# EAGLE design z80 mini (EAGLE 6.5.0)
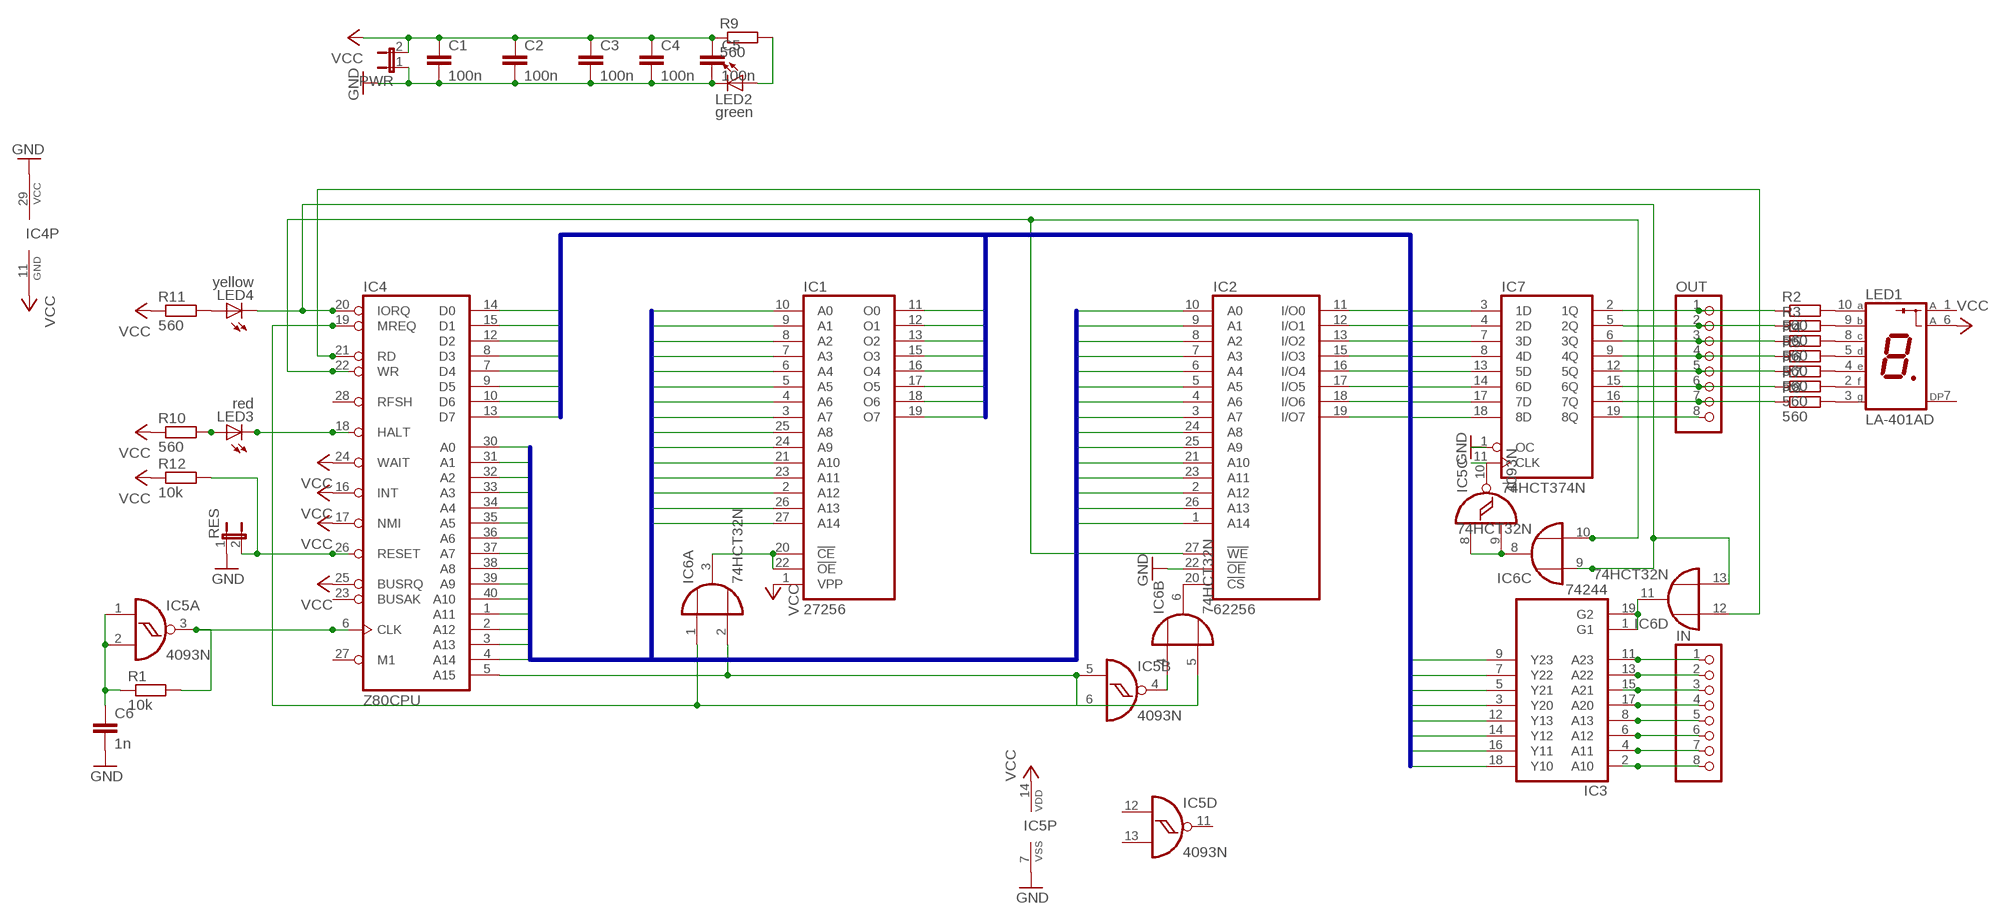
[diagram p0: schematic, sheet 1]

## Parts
C1  100n  C-EU025-025X050  [C025-025X050]
C2  100n  C-EU025-025X050  [C025-025X050]
C3  100n  C-EU025-025X050  [C025-025X050]
C4  100n  C-EU025-025X050  [C025-025X050]
C5  100n  C-EU025-025X050  [C025-025X050]
C6  1n  C-EU025-025X050  [C025-025X050]
IC1  27256  [DIL28]
IC2  62256  [DIL28]
IC3  74244  [DIL20]
IC4  Z80CPU  [DIL40]
IC5  4093N  [DIL14]
IC6  74HCT32N  [DIL14]
IC7  74HCT374N  [DIL20]
IN  PINHD-1X8  [1X08]
LED1  LA-401AD  [LA-401]
LED2  green  LED3MM  [LED3MM]
LED3  red  LED3MM  [LED3MM]
LED4  yellow  LED3MM  [LED3MM]
OUT  PINHD-1X8  [1X08]
PWR  JP1E  [JP1]
R1  10k  R-EU_0204/7  [0204/7]
R2  560  R-EU_0204/7  [0204/7]
R3  560  R-EU_0204/7  [0204/7]
R4  560  R-EU_0204/7  [0204/7]
R5  560  R-EU_0204/7  [0204/7]
R6  560  R-EU_0204/7  [0204/7]
R7  560  R-EU_0204/7  [0204/7]
R8  560  R-EU_0204/7  [0204/7]
R9  560  R-EU_0204/7  [0204/7]
R10  560  R-EU_0204/7  [0204/7]
R11  560  R-EU_0204/7  [0204/7]
R12  10k  R-EU_0204/7  [0204/7]
RES  JP1E  [JP1]

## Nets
A0: IC1.10(A0) IC2.10(A0) IC4.30(A0)
A1: IC1.9(A1) IC2.9(A1) IC4.31(A1)
A2: IC1.8(A2) IC2.8(A2) IC4.32(A2)
A3: IC1.7(A3) IC2.7(A3) IC4.33(A3)
A4: IC1.6(A4) IC2.6(A4) IC4.34(A4)
A5: IC1.5(A5) IC2.5(A5) IC4.35(A5)
A6: IC1.4(A6) IC2.4(A6) IC4.36(A6)
A7: IC1.3(A7) IC2.3(A7) IC4.37(A7)
A8: IC1.25(A8) IC2.24(A8) IC4.38(A8)
A9: IC1.24(A9) IC2.25(A9) IC4.39(A9)
A10: IC1.21(A10) IC2.21(A10) IC4.40(A10)
A11: IC1.23(A11) IC2.23(A11) IC4.1(A11)
A12: IC1.2(A12) IC2.2(A12) IC4.2(A12)
A13: IC1.26(A13) IC2.26(A13) IC4.3(A13)
A14: IC1.27(A14) IC2.1(A14) IC4.4(A14)
D0: IC1.11(O0) IC2.11(I/O0) IC3.18(Y10) IC4.14(D0) IC7.3(1D)
D1: IC1.12(O1) IC2.12(I/O1) IC3.16(Y11) IC4.15(D1) IC7.4(2D)
D2: IC1.13(O2) IC2.13(I/O2) IC3.14(Y12) IC4.12(D2) IC7.7(3D)
D3: IC1.15(O3) IC2.15(I/O3) IC3.12(Y13) IC4.8(D3) IC7.8(4D)
D4: IC1.16(O4) IC2.16(I/O4) IC3.3(Y20) IC4.7(D4) IC7.13(5D)
D5: IC1.17(O5) IC2.17(I/O5) IC3.5(Y21) IC4.9(D5) IC7.14(6D)
D6: IC1.18(O6) IC2.18(I/O6) IC3.7(Y22) IC4.10(D6) IC7.17(7D)
D7: IC1.19(O7) IC2.19(I/O7) IC3.9(Y23) IC4.13(D7) IC7.18(8D)
GND: C1.2 C2.2 C3.2 C4.2 C5.2 C6.2 IC2.22(!OE) IC4.29(VCC) IC5.7(P:VSS) IC7.1(OC) LED2.K(C) PWR.1 RES.1
N$1: C6.1 IC5.1(A:I0) IC5.2(A:I1) R1.1
N$2: IC4.6(CLK) IC5.3(A:O) R1.2
N$3: IC3.11(A23) IN.1
N$4: IC3.13(A22) IN.2
N$5: IC3.15(A21) IN.3
N$6: IC3.17(A20) IN.4
N$7: IC3.8(A13) IN.5
N$8: IC3.6(A12) IN.6
N$9: IC3.4(A11) IN.7
N$10: IC3.2(A10) IN.8
N$11: IC7.2(1Q) OUT.1 R2.1
N$12: IC7.5(2Q) OUT.2 R3.1
N$13: IC7.6(3Q) OUT.3 R4.1
N$14: IC7.9(4Q) OUT.4 R5.1
N$15: IC7.12(5Q) OUT.5 R6.1
N$16: IC7.15(6Q) OUT.6 R7.1
N$17: IC7.16(7Q) OUT.7 R8.1
N$18: IC7.19(8Q) OUT.8
N$19: LED1.10(A) R2.2
N$20: LED1.9(B) R3.2
N$21: LED1.8(C) R4.2
N$22: LED1.5(D) R5.2
N$23: LED1.4(E) R6.2
N$24: LED1.2(F) R7.2
N$25: LED1.3(G) R8.2
N$26: IC5.4(B:O) IC6.4(B:I0)
N$27: IC2.20(!CS) IC6.6(B:O)
N$28: IC1.20(!CE) IC1.22(!OE) IC6.3(A:O)
N$29: IC4.5(A15) IC5.5(B:I0) IC5.6(B:I1) IC6.2(A:I1)
N$30: IC4.19(MREQ) IC6.1(A:I0) IC6.5(B:I1)
N$31: IC2.27(!WE) IC4.22(WR) IC6.10(C:I1)
N$32: IC5.10(C:O) IC7.11(CLK)
N$33: IC5.8(C:I0) IC5.9(C:I1) IC6.8(C:O)
N$34: IC4.20(IORQ) IC6.9(C:I0) IC6.13(D:I1) LED4.K(C)
N$35: IC3.1(G1) IC3.19(G2) IC6.11(D:O)
N$36: IC4.18(HALT) LED3.K(C)
N$37: IC4.21(RD) IC6.12(D:I0)
N$38: LED2.A R9.2
N$39: LED3.A R10.2
N$40: LED4.A R11.2
N$41: IC4.26(RESET) R12.2 RES.2
VCC: C1.1 C2.1 C3.1 C4.1 C5.1 IC1.1(VPP) IC4.11(GND) IC4.16(INT) IC4.17(NMI) IC4.24(WAIT) IC4.25(BUSRQ) IC5.14(P:VDD) LED1.6(A) PWR.2 R9.1 R10.1 R11.1 R12.1
Unconnected: IC4.23(BUSAK) IC4.27(M1) IC4.28(RFSH) IC5.11(D:O) IC5.12(D:I0) IC5.13(D:I1) LED1.1(A) LED1.7(DP)

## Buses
D[0..7]
A[0..14]

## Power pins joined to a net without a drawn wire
GND: IC1.14(GND) IC2.14(GND) IC3.10(GND) IC6.7(P:GND) IC7.10(GND)
VCC: IC1.28(VCC) IC2.28(VCC) IC3.20(VCC) IC6.14(P:VCC) IC7.20(VCC)

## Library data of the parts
C1-C6 = resistor:C-EU: CAPACITOR, European symbol
IC1 = 0RB_Memory:27256: MEMORY
IC2 = 0RB_Memory:62256: 32K*8 SRAM
IC3 = 0RB_TTL:74244: 74244 as one IC
IC4 = 0RB_Zilog:Z80CPU: Z80 CPU
IC5 = 40xx:4093: Quad 2-input NAND schmitt trigger
IC6 = 74xx-eu:74*32: Quad 2-input OR gate
IC7 = 74xx-eu:74*374: Octal D type transparent LATCH, edge triggered
IN OUT = pinhead:PINHD-1X8: PIN HEADER
LED1 = led-7-segment:LA-401*D: Single Digit LED Numeric Display (anode common) Source: ROHM .. la-1401dn.pdf
LED2-LED4 = led:LED: LED
PWR RES = jumper:JP1E: JUMPER
R1-R12 = resistor:R-EU_: RESISTOR, European symbol

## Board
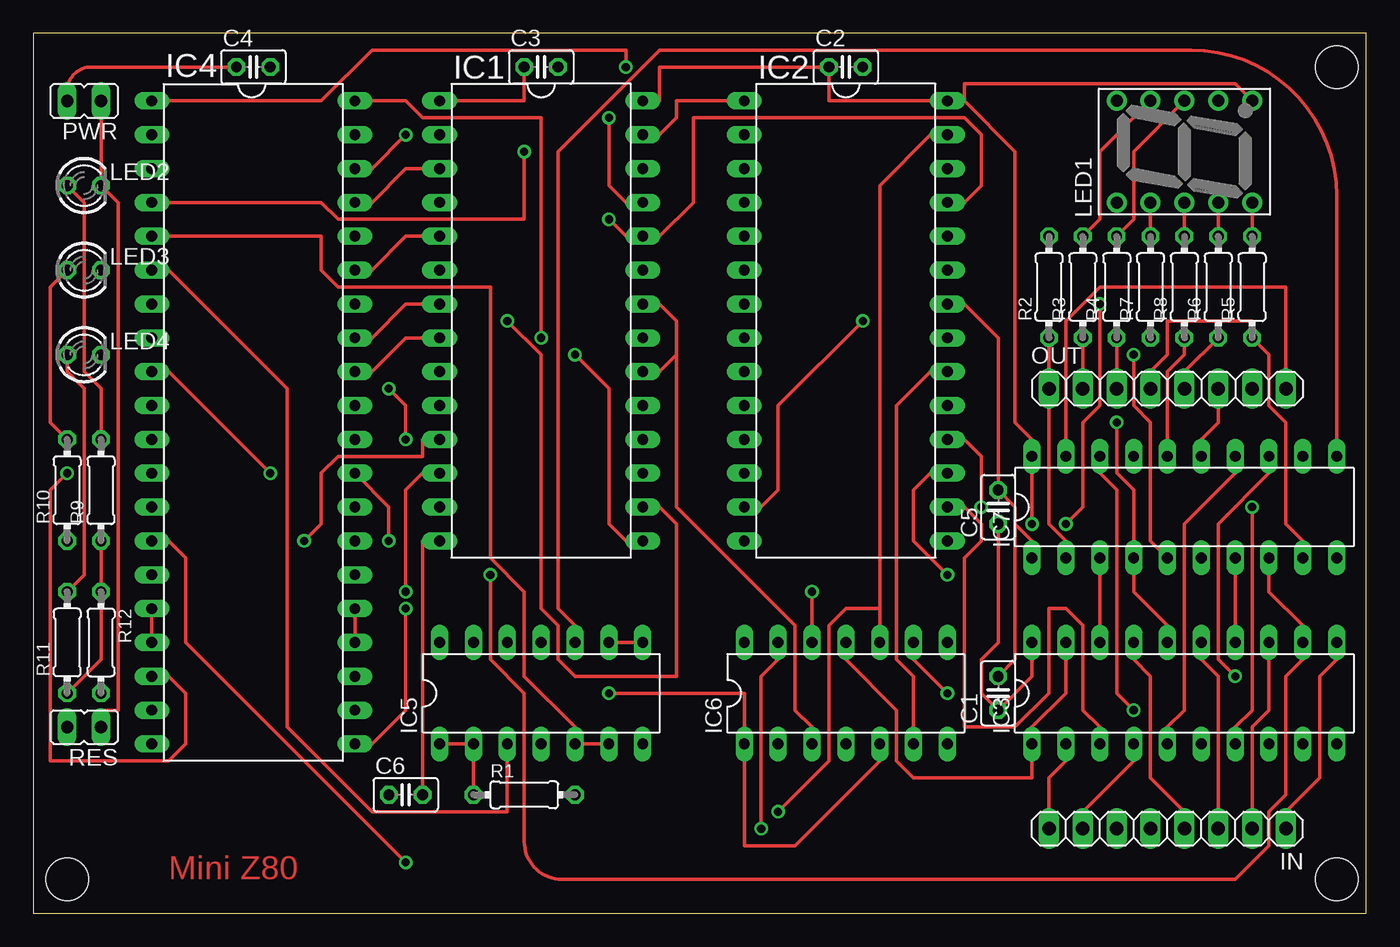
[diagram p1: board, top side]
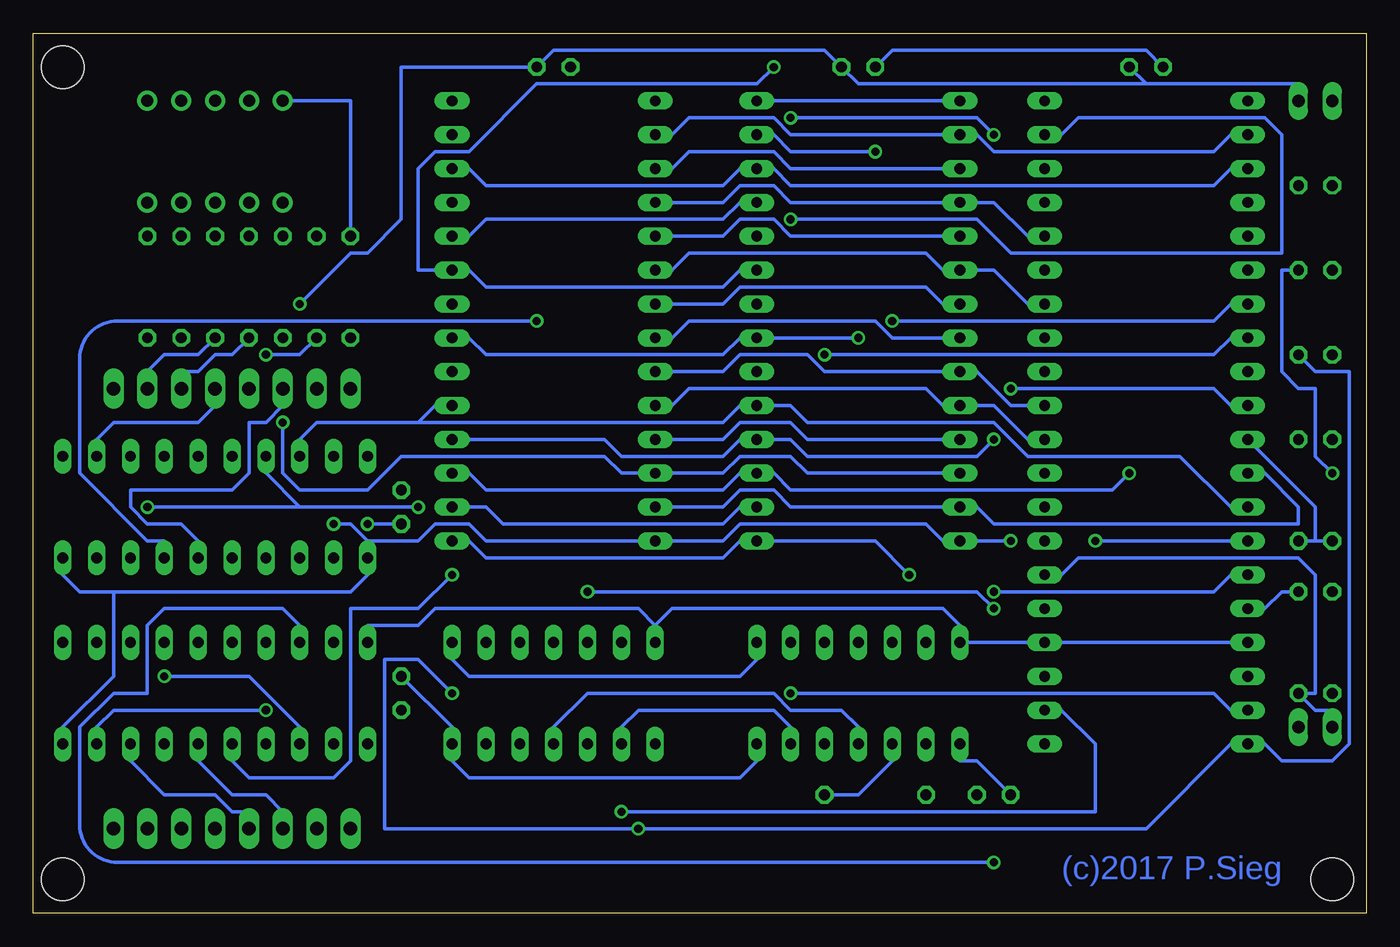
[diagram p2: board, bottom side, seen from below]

Size 100 x 66.03 mm. Coordinates in mm from the lower left corner, seen from the top.
Outline: 0,0 100,0 100,66.03 0,66.03 0,0
Copper layers (1*16): Top 0.035mm / dielectric 1.5mm / Bottom 0.035mm
Design rules "default": minimum track width 10mil, minimum drill 24mil, track to track 8mil, track to pad 8mil, pad to pad 8mil, via to via 8mil, smd to smd 8mil, copper to edge 40mil, drill to drill 8mil, minimum pad ring 10mil, minimum via ring 8mil, stop-mask expansion 4mil, vias tented up to drill 0mil, thermal gap 10mil
Holes 3.2 mm at 2.54,2.54 97.79,63.5 97.79,2.54

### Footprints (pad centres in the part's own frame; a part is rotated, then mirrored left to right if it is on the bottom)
C025-025X050 = drill 0.813 octagon: 1 -1.27,0; 2 1.27,0
DIL28 = drill 0.813 long: 1 -16.51,-7.62; 2 -13.97,-7.62; 3 -11.43,-7.62; 4 -8.89,-7.62; 5 -6.35,-7.62; 6 -3.81,-7.62; 7 -1.27,-7.62; 8 1.27,-7.62; 9 3.81,-7.62; 10 6.35,-7.62; 11 8.89,-7.62; 12 11.43,-7.62; 13 13.97,-7.62; 14 16.51,-7.62; 15 16.51,7.62; 16 13.97,7.62; 17 11.43,7.62; 18 8.89,7.62; 19 6.35,7.62; 20 3.81,7.62; 21 1.27,7.62; 22 -1.27,7.62; 23 -3.81,7.62; 24 -6.35,7.62; 25 -8.89,7.62; 26 -11.43,7.62; 27 -13.97,7.62; 28 -16.51,7.62
DIL20 = drill 0.813 long: 1 -11.43,-3.81; 2 -8.89,-3.81; 3 -6.35,-3.81; 4 -3.81,-3.81; 5 -1.27,-3.81; 6 1.27,-3.81; 7 3.81,-3.81; 8 6.35,-3.81; 9 8.89,-3.81; 10 11.43,-3.81; 11 11.43,3.81; 12 8.89,3.81; 13 6.35,3.81; 14 3.81,3.81; 15 1.27,3.81; 16 -1.27,3.81; 17 -3.81,3.81; 18 -6.35,3.81; 19 -8.89,3.81; 20 -11.43,3.81
DIL40 = drill 0.813 long: 1 -24.13,-7.62; 2 -21.59,-7.62; 3 -19.05,-7.62; 4 -16.51,-7.62; 5 -13.97,-7.62; 6 -11.43,-7.62; 7 -8.89,-7.62; 8 -6.35,-7.62; 9 -3.81,-7.62; 10 -1.27,-7.62; 11 1.27,-7.62; 12 3.81,-7.62; 13 6.35,-7.62; 14 8.89,-7.62; 15 11.43,-7.62; 16 13.97,-7.62; 17 16.51,-7.62; 18 19.05,-7.62; 19 21.59,-7.62; 20 24.13,-7.62; 21 24.13,7.62; 22 21.59,7.62; 23 19.05,7.62; 24 16.51,7.62; 25 13.97,7.62; 26 11.43,7.62; 27 8.89,7.62; 28 6.35,7.62; 29 3.81,7.62; 30 1.27,7.62; 31 -1.27,7.62; 32 -3.81,7.62; 33 -6.35,7.62; 34 -8.89,7.62; 35 -11.43,7.62; 36 -13.97,7.62; 37 -16.51,7.62; 38 -19.05,7.62; 39 -21.59,7.62; 40 -24.13,7.62
DIL14 = drill 0.813 long: 1 -7.62,-3.81; 2 -5.08,-3.81; 3 -2.54,-3.81; 4 0,-3.81; 5 2.54,-3.81; 6 5.08,-3.81; 7 7.62,-3.81; 8 7.62,3.81; 9 5.08,3.81; 10 2.54,3.81; 11 0,3.81; 12 -2.54,3.81; 13 -5.08,3.81; 14 -7.62,3.81
1X08 = drill 1.016 long: 1 -8.89,0; 2 -6.35,0; 3 -3.81,0; 4 -1.27,0; 5 1.27,0; 6 3.81,0; 7 6.35,0; 8 8.89,0
LA-401 = drill 0.9 pad 1.5: 1 -3.81,5.08; 2 -3.81,2.54; 3 -3.81,0; 4 -3.81,-2.54; 5 -3.81,-5.08; 6 3.81,-5.08; 7 3.81,-2.54; 8 3.81,0; 9 3.81,2.54; 10 3.81,5.08
LED3MM = drill 0.813 octagon: A -1.27,0; K 1.27,0
JP1 = drill 0.914 long: 1 0,-1.27; 2 0,1.27
0204/7 = drill 0.813 octagon: 1 -3.81,0; 2 3.81,0

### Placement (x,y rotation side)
C1  72.39,16.51 90 top
C2  60.96,63.5 0 top
C3  38.1,63.5 0 top
C4  16.51,63.5 0 top
C5  72.39,30.48 90 top
C6  27.94,8.89 0 top
IC1  38.1,44.45 270 top
IC2  60.96,44.45 270 top
IC3  86.36,16.51 0 top
IC4  16.51,36.83 270 top
IC5  38.1,16.51 0 top
IC6  60.96,16.51 0 top
IC7  86.36,30.48 0 top
IN  85.09,6.35 180 top
LED1  86.36,57.15 90 top
LED2  3.81,54.61 0 top
LED3  3.81,48.26 0 top
LED4  3.81,41.91 0 top
OUT  85.09,39.37 0 top
PWR  3.81,60.96 90 top
R1  36.83,8.89 0 top
R2  76.2,46.99 90 top
R3  78.74,46.99 90 top
R4  81.28,46.99 90 top
R5  91.44,46.99 90 top
R6  88.9,46.99 90 top
R7  83.82,46.99 90 top
R8  86.36,46.99 90 top
R9  5.08,31.75 90 top
R10  2.54,31.75 90 top
R11  2.54,20.32 90 top
R12  5.08,20.32 270 top
RES  3.81,13.97 90 top

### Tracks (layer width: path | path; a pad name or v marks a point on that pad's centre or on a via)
A0
  Bottom 0.254: IC4.30 25.4,35.56 27.94,38.1 IC1.10 31.75,38.1 33.02,39.37 50.8,39.37 52.07,38.1 IC2.10
A1
  Bottom 0.254: IC4.31 26.67,38.1 29.21,40.64 IC1.9 40.64,40.64 41.91,41.91 46.99,41.91 48.26,40.64 IC2.9
A2
  Top 0.254: IC4.32 25.4,40.64 27.94,43.18 IC1.8
  Bottom 0.254: IC2.8 52.07,43.18 50.8,44.45 36.83,44.45 35.56,43.18 IC1.8
A3
  Top 0.254: IC4.33 25.4,43.18 27.94,45.72 IC1.7
  Bottom 0.254: IC2.7 48.26,45.72 46.99,46.99 33.02,46.99 31.75,45.72 IC1.7
A4
  Bottom 0.254: IC4.34 25.4,45.72 27.94,48.26 IC1.6 31.75,48.26 33.02,49.53 50.8,49.53 52.07,48.26 IC2.6
A5
  Top 0.254: IC4.35 25.4,48.26 27.94,50.8 IC1.5
  Bottom 0.254: IC2.5 48.26,50.8 46.99,52.07 44.45,52.07 43.18,50.8 IC1.5
A6
  Bottom 0.254: IC4.36 25.4,50.8 27.94,53.34 IC1.4 43.18,53.34 44.45,54.61 46.99,54.61 48.26,53.34 IC2.4
A7
  Top 0.254: IC4.37 25.4,53.34 27.94,55.88 IC1.3
  Bottom 0.254: IC2.3 52.07,55.88 50.8,57.15 44.45,57.15 43.18,55.88 IC1.3
A8  (via drill 0.61)
  Top 0.254: v27.94,58.42 25.4,55.88 IC4.38 | v43.18,59.69 43.18,54.61 44.45,53.34 IC1.25
  Bottom 0.254: v27.94,58.42 29.21,59.69 v43.18,59.69 | IC2.24 67.31,50.8 66.04,52.07 48.26,52.07 46.99,53.34 IC1.25
A9  (via drill 0.61)
  Top 0.254: v43.18,52.07 44.45,50.8 IC1.24 46.99,50.8 49.53,53.34 49.53,59.69 69.85,59.69 71.12,58.42 71.12,54.61 69.85,53.34 IC2.25
  Bottom 0.254: v43.18,52.07 29.21,52.07 26.67,49.53 6.35,49.53 6.35,58.42 7.62,59.69 21.59,59.69 22.86,58.42 IC4.39
A10  (via drill 0.61)
  Top 0.254: v38.1,43.18 38.1,59.69 29.21,59.69 27.94,60.96 IC4.40
  Bottom 0.254: IC2.21 67.31,43.18 66.04,41.91 48.26,41.91 46.99,43.18 IC1.21 v38.1,43.18
A11  (via drill 0.61)
  Top 0.254: v44.45,63.5 44.45,64.77 25.4,64.77 21.59,60.96 IC4.1
  Bottom 0.254: IC1.23 46.99,48.26 48.26,46.99 66.04,46.99 67.31,48.26 IC2.23 71.12,48.26 71.12,55.88 69.85,57.15 67.31,57.15 62.23,62.23 45.72,62.23 v44.45,63.5
A12
  Bottom 0.254: IC4.2 10.16,58.42 11.43,57.15 27.94,57.15 29.21,58.42 IC1.2 43.18,58.42 44.45,59.69 50.8,59.69 52.07,58.42 IC2.2
A13
  Bottom 0.254: IC4.3 10.16,55.88 11.43,54.61 43.18,54.61 44.45,55.88 IC1.26 46.99,55.88 48.26,54.61 66.04,54.61 67.31,55.88 IC2.26
A14  (via drill 0.61)
  Top 0.254: v36.83,57.15 36.83,52.07 22.86,52.07 21.59,53.34 IC4.4 | IC2.1 48.26,60.96 48.26,59.69 46.99,58.42 IC1.27
  Bottom 0.254: v36.83,57.15 43.18,57.15 44.45,58.42 IC1.27
D0  (via drill 0.61)
  Top 0.254: IC3.18 IC7.3 | v20.32,27.94 21.59,29.21 21.59,33.02 22.86,34.29 29.21,34.29 29.21,35.56 IC1.11 | v27.94,3.81 11.43,20.32 11.43,26.67 10.16,27.94 IC4.14
  Bottom 0.254: IC4.14 v20.32,27.94 | IC2.11 48.26,35.56 46.99,36.83 43.18,36.83 41.91,35.56 IC1.11 | v27.94,3.81 93.68,3.81 arc90 96.52,6.65 96.52,13.97 93.98,16.51 91.44,16.51 91.44,21.59 90.17,22.86 81.28,22.86 80.01,21.59 IC3.18
D1  (via drill 0.61)
  Top 0.254: IC3.16 85.09,21.59 82.55,24.13 IC7.4 82.55,31.75 81.28,33.02 v81.28,36.83 | v27.94,24.13 27.94,31.75 29.21,33.02 IC1.12
  Bottom 0.254: v27.94,24.13 11.43,24.13 10.16,25.4 IC4.15 | IC1.12 41.91,33.02 43.18,34.29 46.99,34.29 48.26,33.02 IC2.12 55.88,33.02 57.15,34.29 72.39,34.29 74.93,31.75 80.01,31.75 81.28,33.02 v81.28,36.83
D2  (via drill 0.61)
  Top 0.254: IC7.7 IC3.14 | v62.23,44.45 55.88,38.1 55.88,31.75 54.61,30.48 IC2.13
  Bottom 0.254: IC2.13 48.26,30.48 46.99,31.75 44.45,31.75 43.18,30.48 IC1.13 29.21,30.48 27.94,29.21 5.08,29.21 5.08,30.48 7.62,33.02 IC4.12 | v62.23,44.45 93.68,44.45 arc-90 96.52,41.61 96.52,33.02 91.44,27.94 90.17,27.94 IC7.7
D3  (via drill 0.61)
  Top 0.254: IC7.8 92.71,24.13 95.25,21.59 IC3.12 95.25,19.05 93.98,17.78 93.98,8.89 92.71,7.62 92.71,5.08 90.17,2.54 39.67,2.54 arc-90 36.83,5.38 36.83,16.51 34.29,19.05 v34.29,25.4 | v40.64,41.91 43.18,39.37 43.18,29.21 44.45,27.94 IC1.15
  Bottom 0.254: IC2.15 67.31,27.94 66.04,26.67 48.26,26.67 46.99,27.94 IC1.15 36.83,27.94 v34.29,25.4 | v40.64,41.91 11.43,41.91 10.16,43.18 IC4.8
D4  (via drill 0.61)
  Top 0.254: v90.17,17.78 88.9,19.05 88.9,29.21 92.71,33.02 IC7.13 | v35.56,44.45 38.1,41.91 38.1,22.86 39.37,21.59 39.37,19.05 40.64,17.78 48.26,17.78 48.26,29.21 46.99,30.48 IC1.16 | IC3.3 80.01,13.97 78.74,15.24 78.74,21.59 77.47,22.86 76.2,22.86 76.2,16.51 73.66,13.97 69.85,13.97 69.85,26.67 71.12,27.94 71.12,29.21 69.85,30.48 IC2.16
  Bottom 0.254: v90.17,17.78 83.82,17.78 80.01,13.97 IC3.3 | IC1.16 46.99,30.48 48.26,29.21 64.77,29.21 66.04,30.48 IC2.16 | v35.56,44.45 11.43,44.45 10.16,45.72 IC4.7
D5  (via drill 0.61)
  Top 0.254: IC3.5 85.09,13.97 86.36,15.24 86.36,29.21 90.17,33.02 IC7.14 | v17.78,33.02 10.16,40.64 IC4.9 | v68.58,25.4 66.04,27.94 66.04,31.75 67.31,33.02 IC2.17
  Bottom 0.254: IC2.17 67.31,33.02 66.04,31.75 48.26,31.75 46.99,33.02 IC1.17 44.45,33.02 43.18,31.75 19.05,31.75 v17.78,33.02 | v68.58,25.4 71.12,22.86 76.2,22.86 76.2,11.43 77.47,10.16 83.82,10.16 85.09,11.43 IC3.5
D6  (via drill 0.61)
  Top 0.254: v26.67,39.37 27.94,38.1 v27.94,35.56 | v71.12,30.48 71.12,34.29 69.85,35.56 IC2.18 | v91.44,30.48 91.44,15.24 90.17,13.97 IC3.7
  Bottom 0.254: IC2.18 57.15,35.56 55.88,34.29 48.26,34.29 46.99,35.56 IC1.18 43.18,35.56 41.91,34.29 29.21,34.29 v27.94,35.56 | v26.67,39.37 11.43,39.37 10.16,38.1 IC4.10 | 80.01,30.48 82.55,33.02 IC7.17 | v71.12,30.48 80.01,30.48 | 80.01,30.48 v91.44,30.48
D7  (via drill 0.61)
  Top 0.254: v82.55,15.24 81.28,16.51 81.28,31.75 80.01,33.02 IC7.18
  Bottom 0.254: IC4.13 10.16,30.48 13.97,34.29 25.4,34.29 27.94,36.83 41.91,36.83 43.18,38.1 IC1.19 46.99,38.1 48.26,36.83 71.12,36.83 | 71.12,36.83 69.85,38.1 IC2.19 | 71.12,36.83 78.74,36.83 80.01,35.56 IC7.18 | v82.55,15.24 93.98,15.24 95.25,13.97 IC3.9
GND  (via drill 0.61)
  Top 0.254: C6.2 29.21,27.94 IC1.14 | 73.66,29.21 74.93,27.94 IC7.1 | 73.66,29.21 73.66,30.48 C5.2 72.39,43.18 69.85,45.72 IC2.22 | C1.2 73.66,19.05 73.66,29.21 | PWR.1 LED2.K 6.35,53.34 6.35,15.24 5.08,15.24 RES.1 | v77.47,29.21 78.74,30.48 78.74,36.83 80.01,38.1 v80.01,45.72 | IC4.29 26.67,30.48 v26.67,27.94
  Bottom 0.254: IC5.7 45.72,11.43 46.99,10.16 67.31,10.16 68.58,11.43 IC6.7 68.58,13.97 C1.2 | 93.98,24.13 93.98,17.78 97.79,13.97 IC3.10 | 93.98,24.13 96.52,24.13 97.79,25.4 IC7.10 | 93.98,24.13 76.2,24.13 74.93,25.4 IC7.1 74.93,27.94 | 74.93,27.94 71.12,27.94 69.85,29.21 67.31,29.21 66.04,27.94 IC2.14 48.26,27.94 46.99,29.21 33.02,29.21 31.75,27.94 IC1.14 v26.67,27.94 | 16.51,62.23 C4.2 | 16.51,62.23 5.08,62.23 PWR.1 | 16.51,62.23 38.1,62.23 C3.2 40.64,64.77 60.96,64.77 C2.2 72.39,63.5 72.39,52.07 74.93,49.53 76.2,49.53 v80.01,45.72 | 74.93,27.94 76.2,29.21 v77.47,29.21
N$1
  Top 0.254: R1.1 IC5.2 IC5.1
  Bottom 0.254: C6.1 29.21,11.43 30.48,11.43 IC5.1
N$2
  Top 0.254: IC4.6 10.16,48.26 19.05,39.37 19.05,13.97 25.4,7.62 35.56,7.62 IC5.3
  Bottom 0.254: R1.2 38.1,8.89 35.56,11.43 IC5.3
N$3
  Top 0.254: IC3.11 97.79,19.05 96.52,17.78 96.52,10.16 93.98,7.62 IN.1
N$4
  Top 0.254: IC3.13 92.71,15.24 91.44,13.97 IN.2
N$5
  Top 0.254: IC3.15 87.63,19.05 88.9,17.78 IN.3
N$6
  Top 0.254: IC3.17 82.55,19.05 83.82,17.78 83.82,10.16 86.36,7.62 IN.4
N$7
  Bottom 0.254: IC3.8 92.71,11.43 90.17,8.89 86.36,8.89 85.09,7.62 83.82,7.62 IN.5
N$8
  Bottom 0.254: IC3.6 87.63,11.43 85.09,8.89 82.55,8.89 81.28,7.62 IN.6
N$9
  Top 0.254: IC3.4 82.55,11.43 78.74,7.62 IN.7
N$10
  Top 0.254: IC3.2 77.47,11.43 76.2,10.16 IN.8
N$11
  Top 0.254: R2.1 OUT.1 76.2,29.21 77.47,27.94 IC7.2
N$12  (via drill 0.61)
  Top 0.254: OUT.2 R3.1 | IC7.5 83.82,27.94 83.82,36.83 82.55,38.1 v82.55,41.91
  Bottom 0.254: v82.55,41.91 80.01,41.91 R3.1
N$13
  Top 0.254: OUT.3 R4.1
  Bottom 0.254: IC7.6 87.63,27.94 88.9,29.21 91.44,29.21 92.71,30.48 92.71,31.75 85.09,31.75 83.82,33.02 83.82,36.83 82.55,36.83 81.28,38.1 OUT.3
N$14
  Top 0.254: IC7.9 95.25,27.94 93.98,29.21 93.98,36.83 92.71,38.1 92.71,41.91 R5.1 91.44,44.45 85.09,44.45 85.09,41.91 83.82,40.64 OUT.4
N$15
  Top 0.254: R6.1 86.36,40.64 OUT.5
  Bottom 0.254: IC7.12 95.25,35.56 93.98,36.83 87.63,36.83 86.36,38.1 OUT.5
N$16
  Top 0.254: IC7.15 87.63,35.56 88.9,36.83 OUT.6
  Bottom 0.254: R7.1 85.09,41.91 86.36,41.91 87.63,40.64 88.9,40.64 OUT.6
N$17
  Top 0.254: R8.1 86.36,41.91 85.09,40.64 IC7.16
  Bottom 0.254: R8.1 87.63,41.91 90.17,41.91 91.44,40.64 OUT.7
N$18
  Top 0.254: IC7.19 77.47,44.45 80.01,46.99 93.98,46.99 OUT.8
N$19
  Bottom 0.254: R2.2 76.2,60.96 LED1.10
N$20
  Top 0.254: R3.2 80.01,52.07 80.01,57.15 LED1.9
N$21
  Top 0.254: R4.2 82.55,52.07 82.55,57.15 LED1.8
N$22
  Top 0.254: R5.2 LED1.5
N$23
  Top 0.254: R6.2 LED1.4
N$24
  Top 0.254: R7.2 LED1.2
N$25
  Top 0.254: R8.2 LED1.3
N$26
  Bottom 0.254: IC5.4 38.1,13.97 39.37,15.24 43.18,15.24 44.45,16.51 58.42,16.51 60.96,13.97 IC6.4
N$27
  Top 0.254: IC6.6 66.04,17.78 64.77,19.05 64.77,38.1 67.31,40.64 IC2.20
N$28
  Top 0.254: 48.26,41.91 46.99,40.64 IC1.20 | 48.26,41.91 48.26,44.45 46.99,45.72 IC1.22 | 48.26,41.91 48.26,30.48 57.15,21.59 57.15,15.24 58.42,13.97 IC6.3
N$29
  Top 0.254: IC5.6 IC5.5 40.64,13.97 36.83,17.78 36.83,24.13 34.29,26.67 34.29,46.99 22.86,46.99 21.59,48.26 21.59,50.8 IC4.5
  Bottom 0.254: IC6.2 55.88,13.97 54.61,15.24 44.45,15.24 43.18,13.97 IC5.6
N$30  (via drill 0.61)
  Top 0.254: v43.18,16.51 53.34,16.51 IC6.1 53.34,5.08 57.15,5.08 63.5,11.43 IC6.5
  Bottom 0.254: v43.18,16.51 11.43,16.51 10.16,15.24 IC4.19
N$31  (via drill 0.61)
  Top 0.254: v55.88,7.62 59.69,11.43 59.69,21.59 60.96,22.86 63.5,22.86 | 63.5,22.86 IC6.10 | 63.5,22.86 63.5,54.61 67.31,58.42 IC2.27
  Bottom 0.254: v55.88,7.62 20.32,7.62 20.32,12.7 22.86,15.24 IC4.22
N$32
  Top 0.254: IC5.10 40.64,21.59 39.37,22.86 39.37,57.15 46.99,64.77 86.86,64.77 arc-90 97.79,53.84 IC7.11
N$33
  Top 0.254: IC5.9 IC5.8
  Bottom 0.254: IC6.8 68.58,19.05 67.31,17.78 46.99,17.78 45.72,19.05 IC5.8
N$34  (via drill 0.61)
  Top 0.254: v54.61,6.35 54.61,17.78 55.88,19.05 IC6.13 | v68.58,16.51 66.04,19.05 IC6.9
  Bottom 0.254: LED4.K 3.81,40.64 1.27,40.64 1.27,12.7 2.54,11.43 6.35,11.43 7.62,12.7 IC4.20 10.16,12.7 16.51,6.35 v54.61,6.35 73.66,6.35 73.66,19.05 71.12,19.05 v68.58,16.51
N$35
  Top 0.254: IC6.11 60.96,19.05 64.77,15.24 64.77,11.43 66.04,10.16 74.93,10.16 IC3.1 74.93,13.97 77.47,16.51 IC3.19
N$36  (via drill 0.61)
  Top 0.254: v2.54,33.02 1.27,31.75 1.27,11.43 10.16,11.43 11.43,12.7 11.43,16.51 10.16,17.78 IC4.18
  Bottom 0.254: v2.54,33.02 3.81,34.29 3.81,39.37 5.08,39.37 6.35,40.64 6.35,48.26 LED3.K
N$37  (via drill 0.61)
  Top 0.254: v27.94,22.86 27.94,15.24 25.4,12.7 IC4.21 | v58.42,24.13 IC6.12
  Bottom 0.254: v27.94,22.86 29.21,24.13 v58.42,24.13
N$38
  Top 0.254: R9.2 5.08,39.37 3.81,40.64 3.81,53.34 LED2.A
N$39
  Top 0.254: R10.2 1.27,36.83 1.27,46.99 LED3.A
N$40
  Top 0.254: R11.2 3.81,25.4 3.81,39.37 2.54,40.64 LED4.A
N$41
  Bottom 0.254: RES.2 2.54,15.24 3.81,15.24 R12.2 3.81,16.51 3.81,25.4 5.08,26.67 21.59,26.67 22.86,25.4 IC4.26
VCC  (via drill 0.61)
  Top 0.254: IC3.20 74.93,17.78 C1.1 71.12,16.51 71.12,19.05 72.39,20.32 C5.1 | IC4.16 IC4.17 | R11.1 5.08,19.05 R12.1 R9.1 | 69.85,60.96 73.66,57.15 73.66,36.83 74.93,35.56 IC7.20 v74.93,29.21 | C4.1 4.34,63.5 arc90 2.54,61.7 PWR.2 | C3.1 36.83,60.96 IC1.1 | IC1.28 46.99,60.96 46.99,63.5 C2.1 59.69,60.96 IC2.28 69.85,60.96 | LED1.6 90.17,62.23 69.85,62.23 69.85,60.96 | IC4.24 IC4.25
  Bottom 0.254: 53.34,21.59 54.61,22.86 69.85,22.86 71.12,21.59 74.93,21.59 IC3.20 | R9.1 3.81,27.94 | 3.81,27.94 R10.1 | R12.1 6.35,24.13 7.62,22.86 IC4.16 | IC4.17 IC4.24 IC5.14 30.48,21.59 31.75,22.86 52.07,22.86 53.34,21.59 | 53.34,21.59 IC6.14 | IC1.28 IC1.1 | C4.1 16.51,64.77 35.56,64.77 C3.1 | C5.1 v74.93,29.21 | IC4.11 3.81,30.48 3.81,27.94

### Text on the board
Top: Mini Z80
Bottom: (c)2017 P.Sieg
